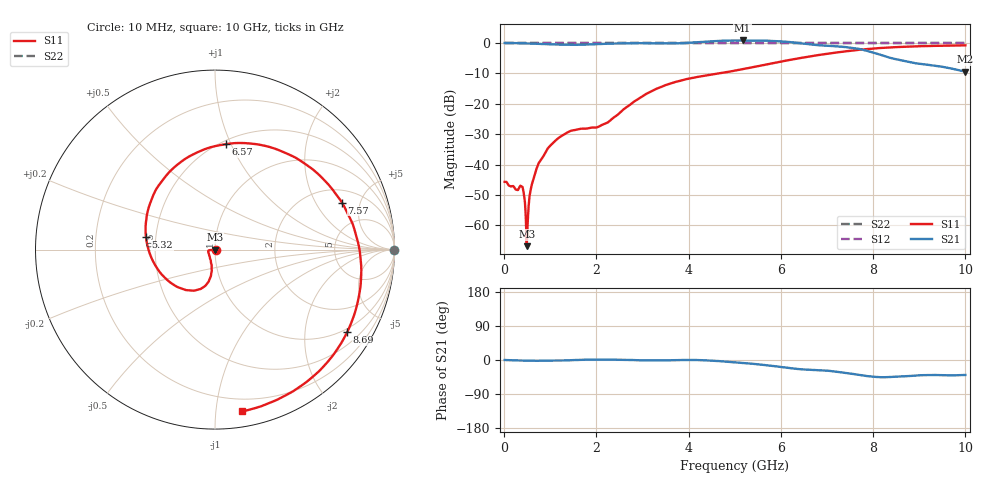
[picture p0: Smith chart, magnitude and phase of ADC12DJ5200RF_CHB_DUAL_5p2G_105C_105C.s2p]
! Texas Instruments, Inc.
! ADC12DJ5200RF - CH B S-Parameters (Dual Ch Mode, Fs = 5.2 GSPS, 105 degC case, 105 degC juntion)
! Port 1 represents the 100-ohm differenal input, Port 2 the digital output
! freq  dbS11  angS11  dbS21 angS21 dbS12 angS12 dbS22 angS22
# HZ S DB R 100
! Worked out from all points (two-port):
!   1000 points, 10 MHz to 10 GHz, reference 100 ohm
!   highest |S21| = 0.84 dB at 5.17 GHz (marker M1); lowest = -9.4 dB at 10 GHz (marker M2)
!   |S21| within 3 dB of the highest: start of sweep to 7.761 GHz
!   lowest |S11| = -66.8 dB at 490 MHz (marker M3), VSWR 1.00, Z = 100 + j0.0909 ohm
!   |S11| at or under -10 dB: start of sweep to 4.655 GHz
!   |S22| runs from 0.0 to 0.0 dB; largest |S21 - S12| = 0.77
!   S11 on the Smith chart (normalised r, x): 10 MHz: 1.01, -0.00; 5.32 GHz: 0.44, +0.07; 6.57 GHz: 0.53, +0.96; 7.57 GHz: 2.79, +3.39; 8.69 GHz: 0.87, -3.26; 10 GHz: 0.11, -1.18
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1e7  -45.69 -2.8  0.00 -0.0  0.00 0.0  0.00 0.0
3.8e8  -47.17 -16.4  -0.07 -1.6  0.00 0.0  0.00 0.0
4.9e8  -66.84 93.5  -0.14 -1.9  0.00 0.0  0.00 0.0
5.2e8  -56.15 -177.4  -0.15 -2.0  0.00 0.0  0.00 0.0
5.8e8  -47.93 -158.5  -0.18 -2.1  0.00 0.0  0.00 0.0
6.5e8  -44.16 -162.0  -0.24 -2.1  0.00 0.0  0.00 0.0
9.2e8  -35.36 -172.3  -0.38 -2.0  0.00 0.0  0.00 0.0
1.25e9  -30.53 -174.5  -0.55 -1.3  0.00 0.0  0.00 0.0
1.68e9  -28.19 -167.0  -0.56 0.4  0.00 0.0  0.00 0.0
2.22e9  -26.31 -127.8  -0.25 0.9  0.00 0.0  0.00 0.0
3.34e9  -14.84 -101.2  -0.11 -1.1  0.00 0.0  0.00 0.0
4.23e9  -11.08 -126.9  0.28 -0.2  0.00 0.0  0.00 0.0
5.01e9  -9.07 -169.7  0.83 -6.4  0.00 0.0  0.00 0.0
5.17e9  -8.62 179.9  0.84 -7.9  0.00 0.0  0.00 0.0
5.32e9  -8.17 169.9  0.81 -9.3  0.00 0.0  0.00 0.0
5.9e9  -6.42 130.4  0.62 -16.9  0.00 0.0  0.00 0.0
6.57e9  -4.57 84.1  -0.36 -25.4  0.00 0.0  0.00 0.0
6.67e9  -4.31 77.3  -0.54 -26.2  0.00 0.0  0.00 0.0
7.57e9  -2.45 20.4  -1.64 -37.0  0.00 0.0  0.00 0.0
8.34e9  -1.48 -18.1  -4.75 -45.0  0.00 0.0  0.00 0.0
8.69e9  -1.23 -32.1  -5.94 -42.7  0.00 0.0  0.00 0.0
1e10  -0.78 -80.5  -9.43 -39.5  0.00 0.0  0.00 0.0
